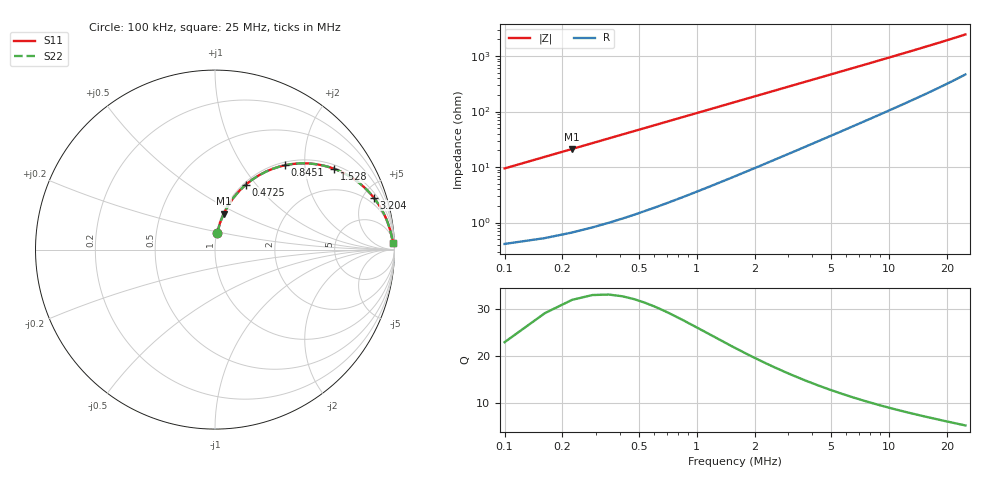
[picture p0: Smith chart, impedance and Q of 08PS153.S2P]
! Coilcraft 0805PS-153 Power Chip Inductor
! 5 February 2003
# MHZ S MA R 50
!Freq  MagS11  AngS11  MagS21  AngS21  MagS12  AngS12  MagS22  AngS22
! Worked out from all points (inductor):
!   403 points, 100 kHz to 25 MHz, reference 50 ohm
!   read as one part in series: L = 15 uH near 224.2 kHz
!   highest Q = 31.9 at 224.2 kHz (marker M1), where L = 15 uH
!   S11 on the Smith chart (normalised r, x): 100 kHz: 1.01, +0.19; 472.5 kHz: 1.03, +0.89; 845.1 kHz: 1.06, +1.58; 1.528 MHz: 1.13, +2.86; 3.204 MHz: 1.38, +5.97; 25 MHz: 10, +48
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0.1  0.09363 82.1  0.9915 -5.4  0.9915 -5.4  0.09363 82.1
0.16209  0.1502 79.4  0.9835 -8.6  0.9835 -8.6  0.1502 79.4
0.22418  0.2052 76.4  0.9723 -11.8  0.9723 -11.8  0.2052 76.4
0.28627  0.2581 73.3  0.9583 -14.9  0.9583 -14.9  0.2581 73.3
0.34836  0.3085 70.3  0.9419 -18.0  0.9419 -18.0  0.3085 70.3
0.47254  0.401 64.6  0.9036 -23.6  0.9036 -23.6  0.401 64.6
0.65881  0.518 56.9  0.8382 -31.2  0.8382 -31.2  0.518 56.9
0.84508  0.6103 50.3  0.7704 -37.6  0.7704 -37.6  0.6103 50.3
1.15553  0.72 41.7  0.6654 -46.0  0.6654 -46.0  0.72 41.7
1.52807  0.8024 34.1  0.5614 -53.3  0.5614 -53.3  0.8024 34.1
1.83852  0.8464 29.5  0.4925 -57.7  0.4925 -57.7  0.8464 29.5
2.21106  0.8818 25.2  0.4269 -61.7  0.4269 -61.7  0.8818 25.2
2.64569  0.9088 21.5  0.3679 -65.1  0.3679 -65.1  0.9088 21.5
3.2045  0.9308 18.1  0.3112 -68.3  0.3112 -68.3  0.9308 18.1
4.26003  0.9535 13.8  0.24 -72.0  0.24 -72.0  0.9535 13.8
6.12273  0.9708 9.8  0.17 -75.3  0.17 -75.3  0.9708 9.8
8.42006  0.9796 7.1  0.1246 -77.0  0.1246 -77.0  0.9796 7.1
10.34485  0.9834 5.8  0.1016 -77.7  0.1016 -77.7  0.9834 5.8
12.58009  0.9861 4.8  0.08348 -78.0  0.08348 -78.0  0.9861 4.8
16.74012  0.9889 3.5  0.06232 -78.0  0.06232 -78.0  0.9889 3.5
20.90015  0.9905 2.8  0.04934 -77.5  0.04934 -77.5  0.9905 2.8
25  0.9915 2.3  0.04061 -76.7  0.04061 -76.7  0.9915 2.3
